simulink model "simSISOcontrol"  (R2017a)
settings: Solver=VariableStepAuto  StartTime=0.0  StopTime=12  RelTol=1e-3
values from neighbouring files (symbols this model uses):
  Kc = 1/k*tau1/(tauc+theta)    [SIMCPI.m]    (also in SIMCPI_nosat.m)
  step_d1 = -2.5    [MISOcontrol.m]    (also in MISO_demo.m; SISOcontrol.m = -2; init.m = 0)
  step_d2 = +2.5    (= 2.5)    [MISOcontrol.m]    (also in MISO_demo.m; SISOcontrol.m = 2; init.m = 0)
  step_ys1 = 5    [MISOcontrol.m]    (also in MISO_demo.m; SISOcontrol.m = 4)
  step_ys2 = -5    [MISOcontrol.m]    (also in MISO_demo.m; SISOcontrol.m = -4)
  stepTime1 = 30    [MISO_demo.m]    (also in SISOcontrol.m = 2)
  stepTime2 = 60    [MISO_demo.m]    (also in SISOcontrol.m = 4)
  stepTime_d1 = 90    [MISOcontrol.m]    (also in MISO_demo.m; SISOcontrol.m = 6; init.m = 0)
  stepTime_d2 = 120    [MISOcontrol.m]    (also in MISO_demo.m; SISOcontrol.m = 8; init.m = 0)
  sys_den = sys_den/sys_den(2)    [SIMCPI.m]    (also in SIMCPI_nosat.m; SISOcontrol.m = cell2mat(sys_tf.den))
  sys_num = sys_num/sys_den(2)    [SIMCPI.m]    (also in SIMCPI_nosat.m; SISOcontrol.m = cell2mat(sys_tf.num))
  tauI = min(tau1,4*(tauc+theta))    [SIMCPI.m]    (also in SIMCPI_nosat.m)
  Ts = 0.1    [identification.m]    (also in MISOcontrol.m; MISO_demo.m; runSteptest.m; SISOcontrol.m)
  y_s0 = 0    [MISOcontrol.m]    (also in MISO_demo.m; SISOcontrol.m = 4)
undefined symbols (not defined in the file or in its folder): Kb
libraries: simulink x1

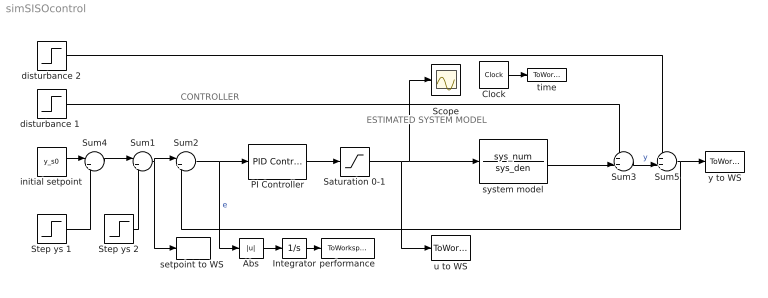
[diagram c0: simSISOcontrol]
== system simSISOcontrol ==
  note: ESTIMATED SYSTEM MODEL
  note: CONTROLLER
  Abs : Abs  ZeroCross=off
  Clock : Clock
  Integrator : Integrator  ZeroCross=off
  PI Controller : simulink/Continuous/PID Controller  Controller=PI  TimeDomain=Continuous-time  SampleTime=-1  IntegratorMethod=Forward Euler  FilterMethod=Forward Euler  Form=Parallel  UseFilter=on  ControllerParametersSource=internal  P=Kc  I=Kc/tauI  D=0  N=100  InitialConditionSource=internal  InitialConditionForIntegrator=0  InitialConditionForFilter=0  ExternalReset=none  LimitOutput=on  UpperSaturationLimit=1  LowerSaturationLimit=0  LinearizeAsGain=on  AntiWindupMode=clamping  Kb=Kb  TrackingMode=off  Kt=1  PParamMin=[]  PParamMax=[]  IParamMin=[]  IParamMax=[]  DParamMin=[]  DParamMax=[]  NParamMin=[]  NParamMax=[]  KbParamMin=[]  KbParamMax=[]  KtParamMin=[]  KtParamMax=[]  POutMin=[]  POutMax=[]  IOutMin=[]  IOutMax=[]  DOutMin=[]  DOutMax=[]  NOutMin=[]  NOutMax=[]  KbOutMin=[]  KbOutMax=[]  KtOutMin=[]  KtOutMax=[]  IntegratorOutMin=[]  IntegratorOutMax=[]  FilterOutMin=[]  FilterOutMax=[]  SumOutMin=[]  SumOutMax=[]  SumI1OutMin=[]  SumI1OutMax=[]  SumI2OutMin=[]  SumI2OutMax=[]  SumI3OutMin=[]  SumI3OutMax=[]  SumDOutMin=[]  SumDOutMax=[]  SaturationOutMin=[]  SaturationOutMax=[]  IntegratorContinuousStateAttributes=''  IntegratorStateMustResolveToSignalObject=off  IntegratorRTWStateStorageClass=Auto  FilterContinuousStateAttributes=''  FilterStateMustResolveToSignalObject=off  FilterRTWStateStorageClass=Auto  DifferentiatorICPrevScaledInput=0  DifferentiatorOutMin=[]  DifferentiatorOutMax=[]  InitialConditionSetting=State (most efficient)
  Saturation 0-1 : Saturate  UpperLimit=1  LowerLimit=0  ZeroCross=off
  Scope : Scope
  Step ys 1 : Step  Time=stepTime1  After=step_ys1  SampleTime=Ts  ZeroCross=off
  Step ys 2 : Step  Time=stepTime2  After=step_ys2  SampleTime=Ts  ZeroCross=off
  Sum1 : Sum  Inputs=|++
  Sum2 : Sum  Inputs=|+-
  Sum3 : Sum  Inputs=++|
  Sum4 : Sum  Inputs=|++
  Sum5 : Sum  Inputs=++|
  "disturbance 1 " : Step  Time=stepTime_d1  After=step_d1  SampleTime=Ts  ZeroCross=off
  disturbance 2 : Step  Time=stepTime_d2  After=step_d2  SampleTime=Ts  ZeroCross=off
  initial setpoint : Constant  Value=y_s0  SampleTime=Ts
  performance : ToWorkspace  VariableName=IAE  SampleTime=Ts
  "setpoint to WS " : ToWorkspace  VariableName=ys  SampleTime=Ts
  system model : TransferFcn  Numerator=sys_num  Denominator=sys_den
  time : ToWorkspace  VariableName=time  SampleTime=Ts
  u to WS : ToWorkspace  VariableName=u  SampleTime=Ts
  y to WS : ToWorkspace  VariableName=y  SampleTime=Ts
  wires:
  system model/1 -> Sum3/2
  Clock/1 -> time/1
  initial setpoint/1 -> Sum4/1
  Sum3/1 -> Sum5/2  "y"
  Sum2/1 -> PI Controller/1, Abs/1  "e"
  Integrator/1 -> performance/1
  Abs/1 -> Integrator/1
  PI Controller/1 -> Saturation 0-1/1
  Saturation 0-1/1 -> Scope/1, system model/1, u to WS/1
  "disturbance 1 "/1 -> Sum3/1
  Sum5/1 -> Sum2/2, y to WS/1
  disturbance 2/1 -> Sum5/1
  Sum1/1 -> Sum2/1, "setpoint to WS "/1
  Sum4/1 -> Sum1/1
  Step ys 1/1 -> Sum4/2
  Step ys 2/1 -> Sum1/2
